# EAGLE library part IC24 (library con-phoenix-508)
PHOENIX
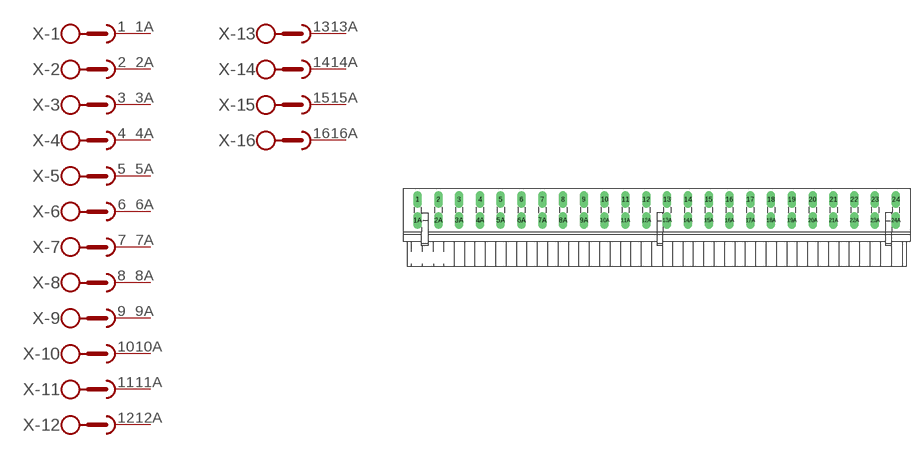
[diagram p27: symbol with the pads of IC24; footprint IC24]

Designator prefix X; gates -1=SKB2 -2=SKB2 -3=SKB2 -4=SKB2 -5=SKB2 -6=SKB2 -7=SKB2 -8=SKB2 -9=SKB2 -10=SKB2 -11=SKB2 -12=SKB2 -13=SKB2 -14=SKB2 -15=SKB2 -16=SKB2 -17=SKB2 -18=SKB2 -19=SKB2 -20=SKB2 -21=SKB2 -22=SKB2 -23=SKB2 -24=SKB2V

## IC24 (OC_FARNELL: unknown; OC_NEWARK: unknown)  [IC24]
1  -1:1  pas
1A  -1:2  pas
2  -2:1  pas
2A  -2:2  pas
3  -3:1  pas
3A  -3:2  pas
4  -4:1  pas
4A  -4:2  pas
5  -5:1  pas
5A  -5:2  pas
6  -6:1  pas
6A  -6:2  pas
7  -7:1  pas
7A  -7:2  pas
8  -8:1  pas
8A  -8:2  pas
9  -9:1  pas
9A  -9:2  pas
10  -10:1  pas
10A  -10:2  pas
11  -11:1  pas
11A  -11:2  pas
12  -12:1  pas
12A  -12:2  pas
13  -13:1  pas
13A  -13:2  pas
14  -14:1  pas
14A  -14:2  pas
15  -15:1  pas
15A  -15:2  pas
16  -16:1  pas
16A  -16:2  pas
17  -17:1  pas
17A  -17:2  pas
18  -18:1  pas
18A  -18:2  pas
19  -19:1  pas
19A  -19:2  pas
20  -20:1  pas
20A  -20:2  pas
21  -21:1  pas
21A  -21:2  pas
22  -22:1  pas
22A  -22:2  pas
23  -23:1  pas
23A  -23:2  pas
24  -24:1  pas
24A  -24:2  pas

## Footprint IC24 (pad centres in mm)
PHOENIX
drill 1.397 long: 1 -58.42,2.54; 1A -58.42,-2.54; 2 -53.34,2.54; 2A -53.34,-2.54; 3 -48.26,2.54; 3A -48.26,-2.54; 4 -43.18,2.54; 4A -43.18,-2.54; 5 -38.1,2.54; 5A -38.1,-2.54; 6 -33.02,2.54; 6A -33.02,-2.54; 7 -27.94,2.54; 7A -27.94,-2.54; 8 -22.86,2.54; 8A -22.86,-2.54; 9 -17.78,2.54; 9A -17.78,-2.54; 10 -12.7,2.54; 10A -12.7,-2.54; 11 -7.62,2.54; 11A -7.62,-2.54; 12 -2.54,2.54; 12A -2.54,-2.54; 13 2.54,2.54; 13A 2.54,-2.54; 14 7.62,2.54; 14A 7.62,-2.54; 15 12.7,2.54; 15A 12.7,-2.54; 16 17.78,2.54; 16A 17.78,-2.54; 17 22.86,2.54; 17A 22.86,-2.54; 18 27.94,2.54; 18A 27.94,-2.54; 19 33.02,2.54; 19A 33.02,-2.54; 20 38.1,2.54; 20A 38.1,-2.54; 21 43.18,2.54; 21A 43.18,-2.54; 22 48.26,2.54; 22A 48.26,-2.54; 23 53.34,2.54; 23A 53.34,-2.54; 24 58.42,2.54; 24A 58.42,-2.54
